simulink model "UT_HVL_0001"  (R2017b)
settings: Solver=FixedStepDiscrete  StartTime=0.0  StopTime=8  FixedStep=0.01  RelTol=1e-3  EnableMultiTasking=on
undefined symbols (not defined in the file): sigbuilder_block

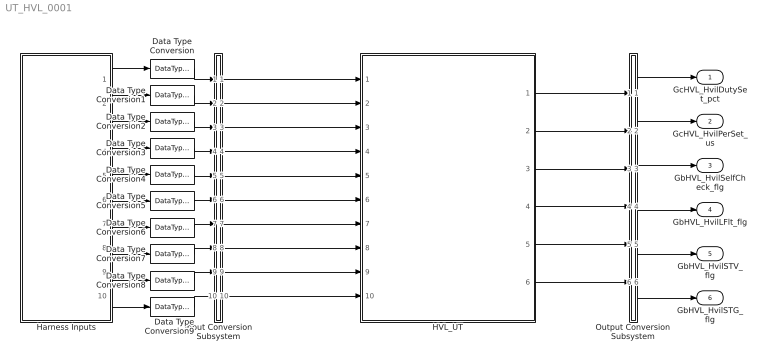
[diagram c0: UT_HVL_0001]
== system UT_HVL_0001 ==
  Data Type Conversion{,1..9} (10 alike) : DataTypeConversion
  HVL_UT : ModelReference  ModelNameDialog=HVL_UT  SimulationMode=Normal  ModelReferenceVersion='M100C100'
  Harness Inputs : Subsystem  Tag=STV Subsys  LoadFcn=sigbuilder_block('load');  StartFcn=sigbuilder_block('start');  StopFcn=sigbuilder_block('stop');  ClipboardFcn=sigbuilder_block('clipboard');  mask(Sigbuilder block){tuvar=[0:10]}
      mask init:
      | if ~strcmp(get_param(bdroot(gcb),'SimulationStatus'),'stopped'),tuvar = sigbuilder_block('maskInit'); end
  Input Conversion Subsystem : Subsystem  Tag=__SLT_ICS__  Description=Signal spec. and routing
  Output Conversion Subsystem : Subsystem  Tag=__SLT_OCS__  Description=Signal spec. and routing
  GcHVL_HvilDutySet_pct : Outport
  GcHVL_HvilPerSet_us : Outport  Port=2
  GbHVL_HvilSelfCheck_flg : Outport  Port=3
  GbHVL_HvilLFlt_flg : Outport  Port=4
  GbHVL_HvilSTV_flg : Outport  Port=5
  GbHVL_HvilSTG_flg : Outport  Port=6
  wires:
  Harness Inputs/1(GeMSM_BMUState_enum) -> Data Type Conversion/1
  Harness Inputs/2(GcLDP_HvilDutyOut_pct) -> Data Type Conversion1/1
  Harness Inputs/3(GcLDP_HvilPerOut_ms) -> Data Type Conversion2/1
  Harness Inputs/4(GcLDP_HvilSt_numb) -> Data Type Conversion3/1
  Harness Inputs/5(GcLDP_HvilDutyFbkt_pct) -> Data Type Conversion4/1
  Harness Inputs/6(GcLDP_HvilPerFbk_ms) -> Data Type Conversion5/1
  Harness Inputs/7(GcLDP_HvilStFbk_numb) -> Data Type Conversion6/1
  Harness Inputs/8(GbISP_TFHvilSTG_flg) -> Data Type Conversion7/1
  Harness Inputs/9(GbISP_TFHvilSTV_flg) -> Data Type Conversion8/1
  Harness Inputs/10(GbISP_TFHvilLFlt_flg) -> Data Type Conversion9/1
  Output Conversion Subsystem/1(Outport_1) -> GcHVL_HvilDutySet_pct/1
  Output Conversion Subsystem/2(Outport_2) -> GcHVL_HvilPerSet_us/1
  Output Conversion Subsystem/3(Outport_3) -> GbHVL_HvilSelfCheck_flg/1
  Output Conversion Subsystem/4(Outport_4) -> GbHVL_HvilLFlt_flg/1
  Output Conversion Subsystem/5(Outport_5) -> GbHVL_HvilSTV_flg/1
  Output Conversion Subsystem/6(Outport_6) -> GbHVL_HvilSTG_flg/1
  Input Conversion Subsystem/1(Outport_1) -> HVL_UT/1
  Input Conversion Subsystem/2(Outport_2) -> HVL_UT/2
  Input Conversion Subsystem/3(Outport_3) -> HVL_UT/3
  Input Conversion Subsystem/4(Outport_4) -> HVL_UT/4
  Input Conversion Subsystem/5(Outport_5) -> HVL_UT/5
  Input Conversion Subsystem/6(Outport_6) -> HVL_UT/6
  Input Conversion Subsystem/7(Outport_7) -> HVL_UT/7
  Input Conversion Subsystem/8(Outport_8) -> HVL_UT/8
  Input Conversion Subsystem/9(Outport_9) -> HVL_UT/9
  Input Conversion Subsystem/10(Outport_10) -> HVL_UT/10
  HVL_UT/1 -> Output Conversion Subsystem/1(Inport_1)
  HVL_UT/2 -> Output Conversion Subsystem/2(Inport_2)
  HVL_UT/3 -> Output Conversion Subsystem/3(Inport_3)
  HVL_UT/4 -> Output Conversion Subsystem/4(Inport_4)
  HVL_UT/5 -> Output Conversion Subsystem/5(Inport_5)
  HVL_UT/6 -> Output Conversion Subsystem/6(Inport_6)
  Data Type Conversion/1 -> Input Conversion Subsystem/1(Inport_1)
  Data Type Conversion1/1 -> Input Conversion Subsystem/2(Inport_2)
  Data Type Conversion2/1 -> Input Conversion Subsystem/3(Inport_3)
  Data Type Conversion3/1 -> Input Conversion Subsystem/4(Inport_4)
  Data Type Conversion4/1 -> Input Conversion Subsystem/5(Inport_5)
  Data Type Conversion5/1 -> Input Conversion Subsystem/6(Inport_6)
  Data Type Conversion6/1 -> Input Conversion Subsystem/7(Inport_7)
  Data Type Conversion7/1 -> Input Conversion Subsystem/8(Inport_8)
  Data Type Conversion8/1 -> Input Conversion Subsystem/9(Inport_9)
  Data Type Conversion9/1 -> Input Conversion Subsystem/10(Inport_10)

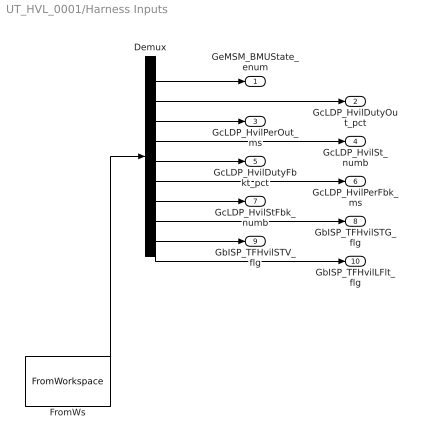
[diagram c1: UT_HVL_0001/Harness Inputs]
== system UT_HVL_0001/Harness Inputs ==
  Demux : Demux  Tag=STV Demux  Outputs=10
  FromWs : FromWorkspace  Tag=STV FromWs  VariableName=tuvar  SampleTime=0
  GeMSM_BMUState_enum : Outport  Tag=STV Outport
  GcLDP_HvilDutyOut_pct : Outport  Tag=STV Outport  Port=2
  GcLDP_HvilPerOut_ms : Outport  Tag=STV Outport  Port=3
  GcLDP_HvilSt_numb : Outport  Tag=STV Outport  Port=4
  GcLDP_HvilDutyFbkt_pct : Outport  Tag=STV Outport  Port=5
  GcLDP_HvilPerFbk_ms : Outport  Tag=STV Outport  Port=6
  GcLDP_HvilStFbk_numb : Outport  Tag=STV Outport  Port=7
  GbISP_TFHvilSTG_flg : Outport  Tag=STV Outport  Port=8
  GbISP_TFHvilSTV_flg : Outport  Tag=STV Outport  Port=9
  GbISP_TFHvilLFlt_flg : Outport  Tag=STV Outport  Port=10
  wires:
  FromWs/1 -> Demux/1
  Demux/1 -> GeMSM_BMUState_enum/1
  Demux/2 -> GcLDP_HvilDutyOut_pct/1
  Demux/3 -> GcLDP_HvilPerOut_ms/1
  Demux/4 -> GcLDP_HvilSt_numb/1
  Demux/5 -> GcLDP_HvilDutyFbkt_pct/1
  Demux/6 -> GcLDP_HvilPerFbk_ms/1
  Demux/7 -> GcLDP_HvilStFbk_numb/1
  Demux/8 -> GbISP_TFHvilSTG_flg/1
  Demux/9 -> GbISP_TFHvilSTV_flg/1
  Demux/10 -> GbISP_TFHvilLFlt_flg/1

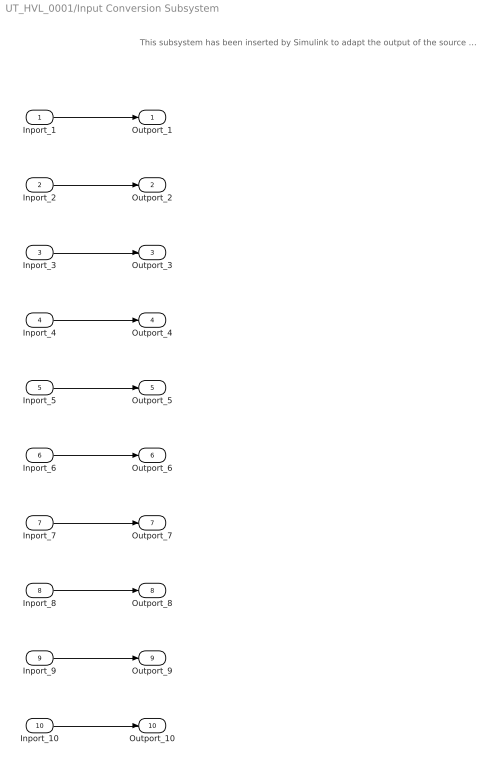
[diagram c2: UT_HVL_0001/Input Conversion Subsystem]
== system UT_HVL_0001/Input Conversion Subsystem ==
  note: This subsystem has been inserted by Simulink to adapt the output of the source blocks to the interface required by the harnessed component. Modifying the contents of this subsystem may result in compilation and simulation failure.
  Inport_1 : Inport
  Inport_2 : Inport  Port=2
  Inport_3 : Inport  Port=3
  Inport_4 : Inport  Port=4
  Inport_5 : Inport  Port=5
  Inport_6 : Inport  Port=6
  Inport_7 : Inport  Port=7
  Inport_8 : Inport  Port=8
  Inport_9 : Inport  Port=9
  Inport_10 : Inport  Port=10
  Outport_1 : Outport
  Outport_2 : Outport  Port=2
  Outport_3 : Outport  Port=3
  Outport_4 : Outport  Port=4
  Outport_5 : Outport  Port=5
  Outport_6 : Outport  Port=6
  Outport_7 : Outport  Port=7
  Outport_8 : Outport  Port=8
  Outport_9 : Outport  Port=9
  Outport_10 : Outport  Port=10
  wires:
  Inport_1/1 -> Outport_1/1
  Inport_2/1 -> Outport_2/1
  Inport_3/1 -> Outport_3/1
  Inport_4/1 -> Outport_4/1
  Inport_5/1 -> Outport_5/1
  Inport_6/1 -> Outport_6/1
  Inport_7/1 -> Outport_7/1
  Inport_8/1 -> Outport_8/1
  Inport_9/1 -> Outport_9/1
  Inport_10/1 -> Outport_10/1

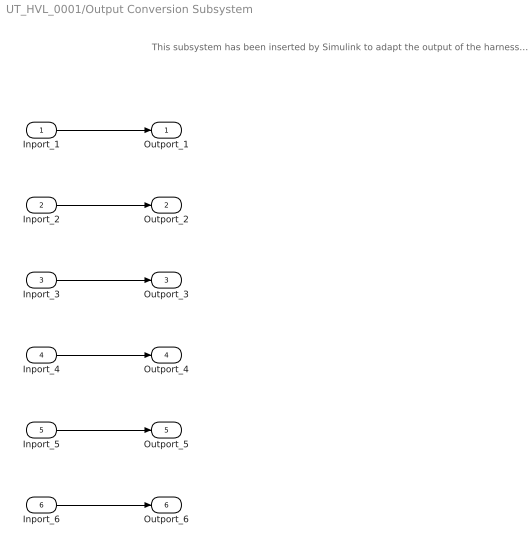
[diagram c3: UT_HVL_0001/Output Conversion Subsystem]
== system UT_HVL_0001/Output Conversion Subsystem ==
  note: This subsystem has been inserted by Simulink to adapt the output of the harnessed component to the interface required by the sink blocks. Modifying the contents of this subsystem may result in compilation and simulation failure.
  Inport_1 : Inport
  Inport_2 : Inport  Port=2
  Inport_3 : Inport  Port=3
  Inport_4 : Inport  Port=4
  Inport_5 : Inport  Port=5
  Inport_6 : Inport  Port=6
  Outport_1 : Outport
  Outport_2 : Outport  Port=2
  Outport_3 : Outport  Port=3
  Outport_4 : Outport  Port=4
  Outport_5 : Outport  Port=5
  Outport_6 : Outport  Port=6
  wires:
  Inport_1/1 -> Outport_1/1
  Inport_2/1 -> Outport_2/1
  Inport_3/1 -> Outport_3/1
  Inport_4/1 -> Outport_4/1
  Inport_5/1 -> Outport_5/1
  Inport_6/1 -> Outport_6/1
